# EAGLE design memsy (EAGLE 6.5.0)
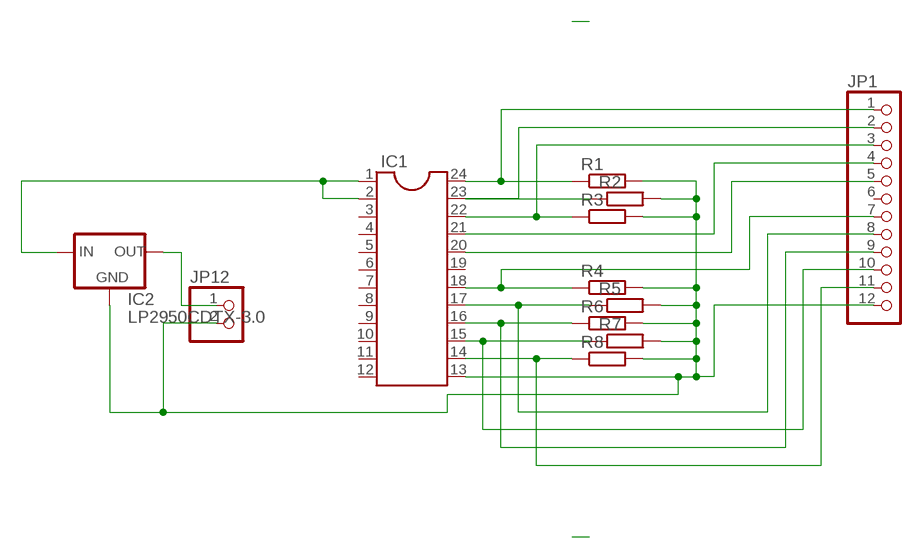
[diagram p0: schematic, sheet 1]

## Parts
IC1  DIL24-6  [DIL24-6]
IC2  LP2950CDTX-3.0  [DPACK]
JP1  PINHD-1X12  [1X12]
JP12  PINHD-1X2  [1X02]
R1  R-EU_R0805  [R0805]
R2  R-EU_R0805  [R0805]
R3  R-EU_R0805  [R0805]
R4  R-EU_R0805  [R0805]
R5  R-EU_R0805  [R0805]
R6  R-EU_R0805  [R0805]
R7  R-EU_R0805  [R0805]
R8  R-EU_R0805  [R0805]

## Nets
N$1: IC1.24 JP1.1 R1.1
N$2: IC1.23 JP1.2 R2.1
N$3: IC1.22 JP1.3 R3.1
N$4: IC1.18 JP1.7 R4.1
N$5: IC1.17 JP1.8 R5.1
N$6: IC1.16 JP1.9 R6.1
N$7: IC1.15 JP1.10 R7.1
N$8: IC1.14 JP1.11 R8.1
N$9: IC1.13 IC2.4(GND) JP1.12 JP12.2 R1.2 R2.2 R3.2 R4.2 R5.2 R6.2 R7.2 R8.2
N$11: IC1.1 IC1.2 IC2.1(IN)
N$13: IC2.3(OUT) JP12.1
N$14: IC1.21 JP1.4
N$15: IC1.20 JP1.5
Unconnected: IC1.3 IC1.4 IC1.5 IC1.6 IC1.7 IC1.8 IC1.9 IC1.10 IC1.11 IC1.12 IC1.19 JP1.6

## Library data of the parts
IC1 = ic-package:DIL24: Dual In Line
IC2 = v-reg:LP2950?*: Source: http://cache.national.com/ds/LP/LP2950.pdf
JP1 = pinhead:PINHD-1X12: PIN HEADER
JP12 = pinhead:PINHD-1X2: PIN HEADER
R1-R8 = rcl:R-EU_: RESISTOR, European symbol

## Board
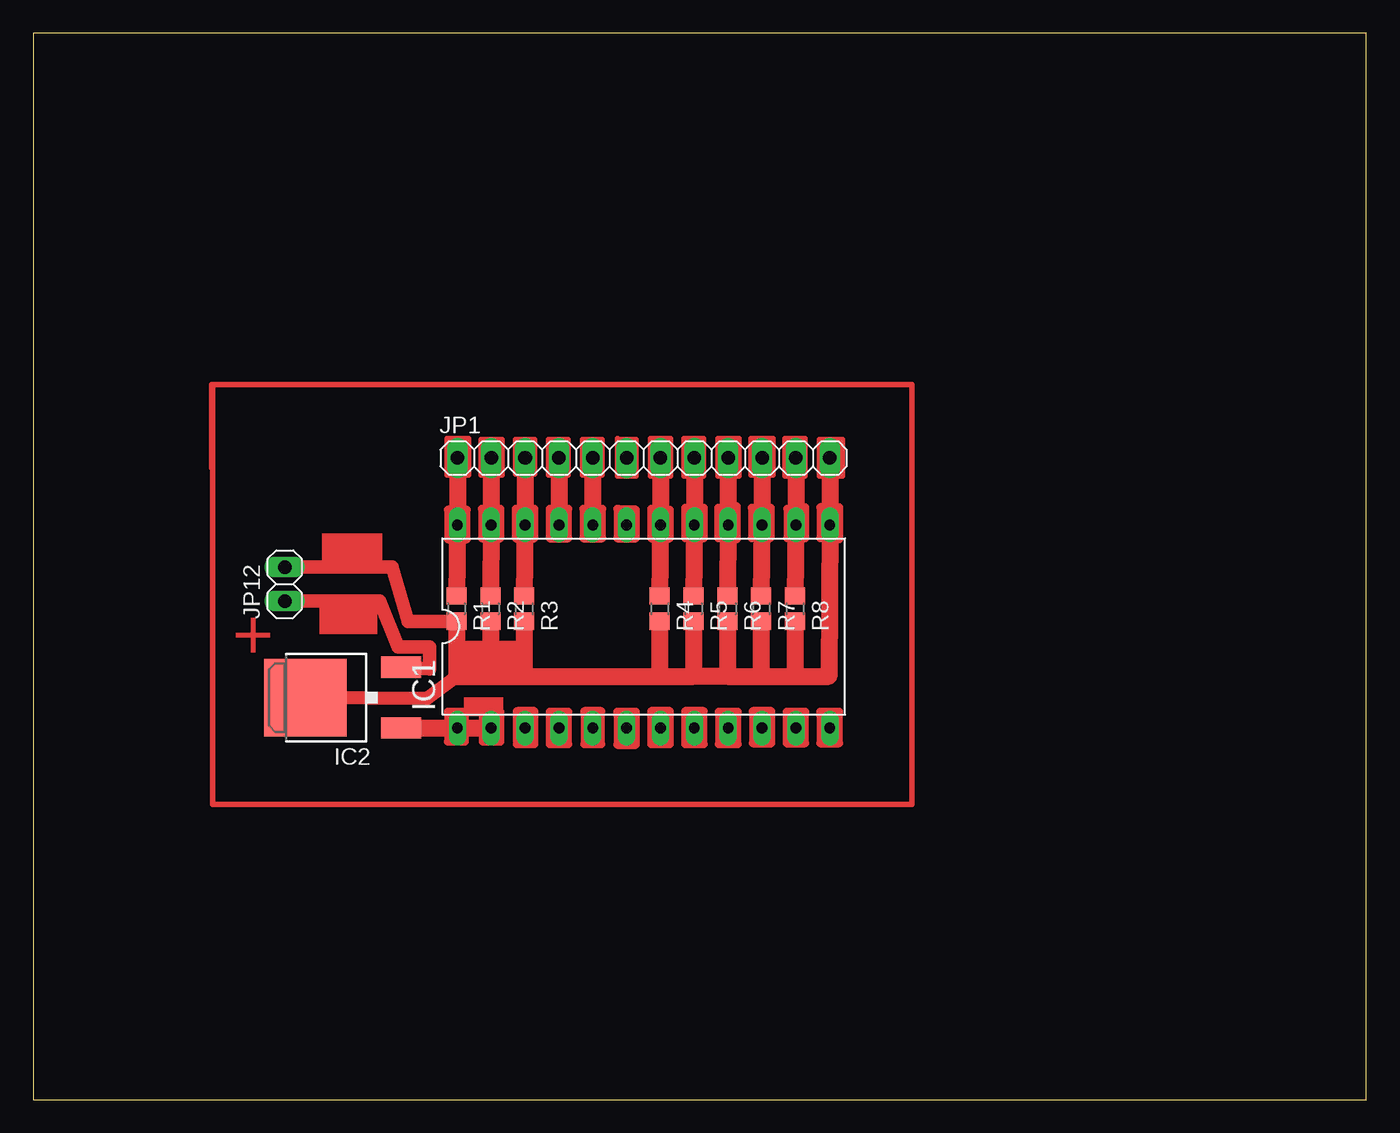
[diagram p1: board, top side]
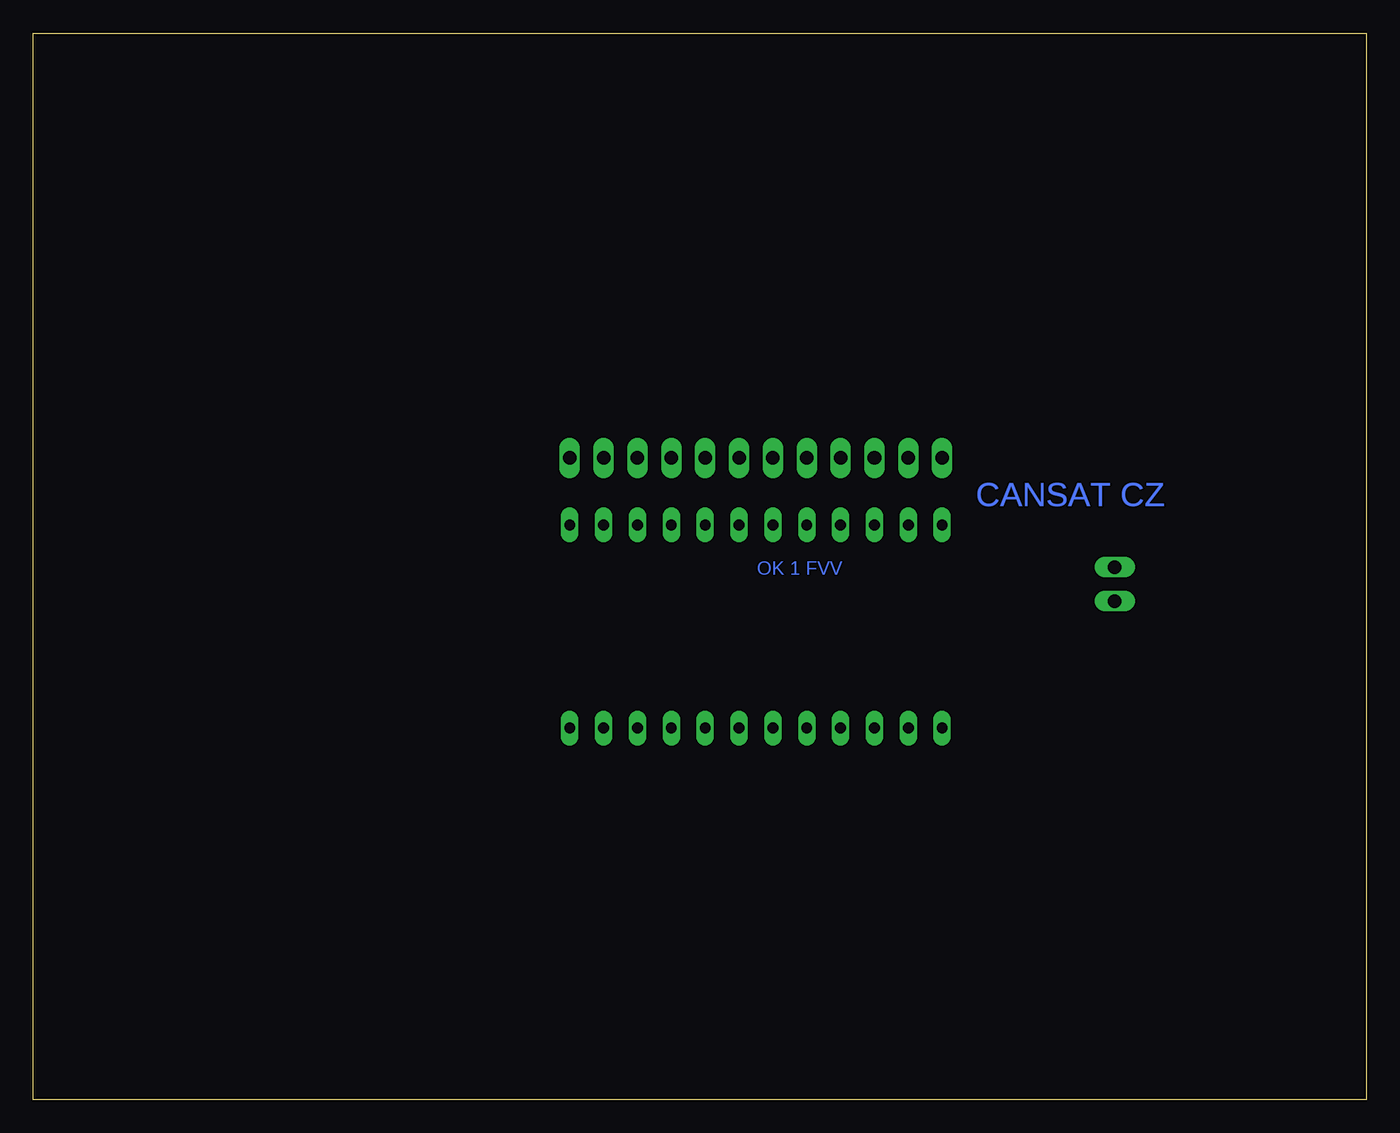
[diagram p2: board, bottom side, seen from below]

Size 100 x 80 mm. Coordinates in mm from the lower left corner, seen from the top.
Outline: 0,0 100,0 100,80 0,80 0,0
Copper layers (1*16): Top 0.035mm / dielectric 1.5mm / Bottom 0.035mm
Design rules "default": minimum track width 10mil, minimum drill 24mil, track to track 8mil, track to pad 8mil, pad to pad 8mil, via to via 8mil, smd to smd 8mil, copper to edge 40mil, drill to drill 8mil, minimum pad ring 10mil, minimum via ring 8mil, stop-mask expansion 4mil, vias tented up to drill 0mil, thermal gap 10mil

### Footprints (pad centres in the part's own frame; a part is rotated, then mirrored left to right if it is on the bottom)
DIL24-6 = drill 0.813 long: 1 -13.97,-7.62; 2 -11.43,-7.62; 3 -8.89,-7.62; 4 -6.35,-7.62; 5 -3.81,-7.62; 6 -1.27,-7.62; 7 1.27,-7.62; 8 3.81,-7.62; 9 6.35,-7.62; 10 8.89,-7.62; 11 11.43,-7.62; 12 13.97,-7.62; 13 13.97,7.62; 14 11.43,7.62; 15 8.89,7.62; 16 6.35,7.62; 17 3.81,7.62; 18 1.27,7.62; 19 -1.27,7.62; 20 -3.81,7.62; 21 -6.35,7.62; 22 -8.89,7.62; 23 -11.43,7.62; 24 -13.97,7.62
DPACK = smd 1.6 x 3: 1 -2.28,-4.8; 3 2.28,-4.8 | smd 5.8 x 6.2: 4 0,2.38
1X12 = drill 1.016 long: 1 -13.97,0; 2 -11.43,0; 3 -8.89,0; 4 -6.35,0; 5 -3.81,0; 6 -1.27,0; 7 1.27,0; 8 3.81,0; 9 6.35,0; 10 8.89,0; 11 11.43,0; 12 13.97,0
1X02 = drill 1.016 long: 1 -1.27,0; 2 1.27,0
R0805 = smd 1.3 x 1.5: 1 -0.95,0; 2 0.95,0

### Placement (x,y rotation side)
IC1  45.78,35.5 0 top
IC2  22.8,30.16 90 top
JP1  45.78,48.13 0 top
JP12  18.86,38.67 90 top
R1  31.75,36.83 270 top
R2  34.29,36.83 270 top
R3  36.83,36.83 270 top
R4  46.99,36.83 270 top
R5  49.53,36.83 270 top
R6  52.07,36.83 270 top
R7  54.61,36.83 270 top
R8  57.15,36.83 270 top

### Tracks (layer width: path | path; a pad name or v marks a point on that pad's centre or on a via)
N$1
  Top 1.27: JP1.1 IC1.24 R1.1
N$2
  Top 1.27: JP1.2 IC1.23 R2.1
N$3
  Top 1.27: JP1.3 IC1.22 R3.1
N$4
  Top 1.27: JP1.7 IC1.18 R4.1
N$5
  Top 1.27: R5.1 IC1.17 JP1.8
N$6
  Top 1.27: R6.1 IC1.16 JP1.9
N$7
  Top 1.27: R7.1 IC1.15 JP1.10
N$8
  Top 1.27: R8.1 IC1.14 JP1.11
N$9
  Top 1.016: 31.75,31.75 29.53,30.1 IC2.4 | R1.2 28.13,35.88 26.92,39.94 JP12.2
  Top 1.27: R1.2 31.75,31.75 34.29,31.75 | 34.29,31.75 36.83,31.75 | 36.83,31.75 46.99,31.75 | 46.99,31.75 49.53,31.75 | 52.07,31.75 54.61,31.75 | 54.61,31.75 57.15,31.75 | R8.2 57.15,31.75 | 57.15,31.75 59.69,31.75 IC1.13 JP1.12 | R7.2 54.61,31.75 | R6.2 52.07,31.75 | R5.2 49.53,31.75 | R4.2 46.99,31.75 | R2.2 34.29,31.75 | R3.2 36.83,31.75 | 52.07,31.75 49.53,31.75
N$11
  Top 1.27: IC2.1 IC1.1 IC1.2
N$13
  Top 1.016: IC2.3 29.72,32.32 29.72,33.97 27.37,33.97 25.97,37.4 JP12.1
N$14
  Top 1.27: JP1.4 IC1.21
N$15
  Top 1.27: JP1.5 IC1.20
N$16
  Top 0.61: 31.11,29.02 31.11,26.86 32.38,26.86 32.38,29.08 31.11,29.08 31.11,29.02
N$17
  Top 0.61: 33.72,29.08 33.72,26.86 35.05,26.86 35.05,29.08 33.78,29.08 33.78,28.96
N$18
  Top 0.61: 36.26,29.15 36.26,26.92
N$19
  Top 0.61: 36.26,26.67 37.59,26.67 37.59,29.15 36.32,29.15 36.32,29.02
N$20
  Top 0.61: 38.73,29.02 38.73,26.67 40.13,26.67 40.13,29.08 38.73,29.08 38.73,29.02
N$21
  Top 0.61: 41.34,29.08 41.34,26.67 42.61,26.67 42.61,29.15 41.34,29.15 41.34,29.08
N$22
  Top 0.61: 43.88,29.08 43.81,29.08 43.81,28.89 43.81,26.61 45.21,26.61 45.21,29.08 43.88,29.08
N$23
  Top 0.61: 46.42,29.15 46.35,29.15 46.35,26.67 47.75,26.67 47.75,29.15 46.42,29.15 | 46.42,29.15 46.42,28.83
N$24
  Top 0.61: 48.96,29.15 48.9,29.15 48.9,26.67 50.29,26.67 50.29,29.15 48.96,29.15 | 48.96,29.15 48.96,28.77
N$25
  Top 0.61: 51.44,29.08 51.44,26.67 52.83,26.67 52.83,29.08 51.5,29.08 51.5,28.83
N$26
  Top 0.61: 54.04,29.15 53.98,29.15 53.98,28.89 53.98,26.73 55.37,26.73 55.37,29.15 54.04,29.15
N$27
  Top 0.61: 56.58,29.08 56.52,29.08 56.52,26.73 57.91,26.73 57.91,29.08 56.58,29.08 | 56.58,29.08 56.58,28.96
N$28
  Top 0.61: 59.12,29.08 59.05,29.08 59.05,28.83 59.05,26.73 60.45,26.73 60.45,29.08 59.12,29.08
N$29
  Top 0.61: 31.18,44.26 31.11,44.26 31.11,42.04 32.51,42.04 32.51,44.26 31.18,44.26 | 31.18,44.26 31.18,44.07
N$30
  Top 0.61: 33.66,44.32 33.66,42.1 35.05,42.1 35.05,44.32 33.78,44.32 33.78,44.2
N$31
  Top 0.61: 36.26,44.32 36.2,44.32 36.2,42.1 37.59,42.1 37.59,44.32
N$32
  Top 0.61: 38.73,44.32 38.73,42.1 40.13,42.1 40.13,44.32
N$33
  Top 0.61: 41.34,44.32 41.27,44.32 41.27,42.1 42.67,42.1 42.67,44.32
N$34
  Top 0.61: 43.88,44.32 43.81,44.32 43.81,42.1 45.21,42.1 45.21,44.26 43.94,44.26 43.94,44.2
N$35
  Top 0.61: 46.42,44.32 46.35,44.32 46.35,42.1 47.75,42.1 47.75,44.26
N$36
  Top 0.61: 48.96,44.39 48.9,44.39 48.9,42.1
N$37
  Top 0.61: 50.1,44.39 50.29,44.39 50.29,42.1
N$38
  Top 0.61: 51.44,44.39 51.37,44.39 51.37,42.1
N$39
  Top 0.61: 52.64,44.51 52.77,44.51 52.77,42.04
N$40
  Top 0.61: 54.04,44.39 53.91,44.39 53.91,42.1
N$41
  Top 0.61: 55.18,44.39 55.31,44.39 55.31,42.16
N$42
  Top 0.61: 56.58,44.32 56.58,42.1
N$43
  Top 0.61: 57.85,44.45 57.91,44.45 57.91,42.1
N$44
  Top 0.61: 59.12,44.45 59.05,44.45 59.05,42.1
N$45
  Top 0.61: 60.33,44.45 60.45,44.45 60.45,42.04
N$46
  Top 0.406: 31.05,49.53 31.05,46.86 32.64,46.86 32.64,49.59 31.05,49.59 31.05,49.53
N$47
  Top 0.406: 33.59,49.47 33.59,49.53 35.18,49.53 35.18,49.47 | 33.59,49.47 33.59,46.86 35.18,46.86 35.18,49.47 | 34.99,49.47 33.59,49.47 | 35.18,49.47 34.99,49.47 | 34.99,49.47 34.99,48.77
N$48
  Top 0.406: 36.2,49.47 36.2,46.93 37.59,46.93 37.59,49.34 37.59,49.47 | 37.59,49.47 36.2,49.47 | 36.2,49.47 36.2,49.53 37.59,49.53 37.59,49.47
N$49
  Top 0.406: 38.67,49.4 38.67,46.86 40.13,46.86 40.13,49.53 38.67,49.53 38.67,49.4
N$50
  Top 0.406: 41.21,49.34 41.21,46.86 42.67,46.86 42.67,49.53 41.21,49.53 41.21,49.34
N$51
  Top 0.406: 43.81,49.59 43.81,49.53 | 43.81,49.53 45.21,49.53 45.21,46.8 43.81,46.8 43.81,49.4 43.81,49.53
N$52
  Top 0.406: 46.35,49.59 46.29,49.59 46.29,49.21 46.29,46.8 47.82,46.8 47.82,49.59 46.35,49.59
N$54
  Top 0.406: 48.83,46.8 50.29,46.8 50.29,49.59 48.83,49.59 48.83,49.28 48.83,49.21 48.83,46.86
N$56
  Top 0.406: 51.37,49.34 51.37,46.8 52.96,46.8 52.96,49.59 51.37,49.59 51.37,49.34 | 51.37,49.34 51.5,49.34
N$57
  Top 0.406: 53.85,49.47 53.85,46.86 55.5,46.86 55.5,49.59 53.85,49.59 53.85,49.47
N$58
  Top 0.406: 56.52,49.59 56.39,49.59 56.39,49.34 56.39,46.8 57.91,46.8 57.91,49.59 56.52,49.59
N$59
  Top 0.406: 58.99,49.53 58.99,46.8 60.71,46.8 60.71,49.53 59.05,49.53 59.05,49.28
N$60
  Top 0.406: 60.01,49.34 60.45,49.34 60.45,49.09
N$61
  Top 0.406: 13.46,53.34 13.46,53.09 13.46,22.16 65.91,22.16 65.91,53.66 13.4,53.66 13.4,47.37
(copper drawn outside any net)
  shapes: Top area x7

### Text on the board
Top: +
Bottom: CANSAT CZ | CANSAT CZ | OK 1 FVV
